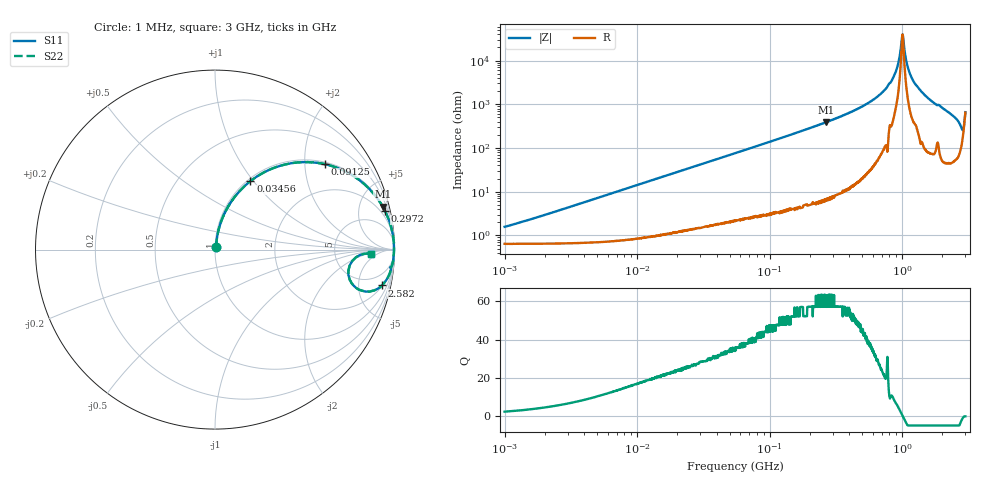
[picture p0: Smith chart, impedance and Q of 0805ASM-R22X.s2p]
!s-Parameter Generated by FASTRON Sdn. Bhd.
!FASTRON P/N : 0805ASM-R22X
!Keysight Technologies: E4991B_MY54100416_A.01.15
!Date: Fri Jun 19 14:51:07 2026
!Version  :Rev00  Fri Jun 19 14:51:07 2026
!Data & Calibration Information:
!Freq  S11  S21  S12  S22
!PortZ  Port1:50+j0  Port2:50+j0
!When reading reference impedance value at option line is always used.
! Remarks : This data is being provided solely for informational purposes.
# Hz S dB R 50
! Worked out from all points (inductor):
!   1601 points, 1 MHz to 3 GHz, reference 50 ohm
!   read as one part in series: L = 228 nH near 1.35 MHz
!   highest Q = 63.3 at 267.6 MHz (marker M1), where L = 234 nH
!   self-resonance near 1.003 GHz
!   S11 on the Smith chart (normalised r, x): 1 MHz: 1.01, +0.03; 34.56 MHz: 1.03, +0.96; 91.25 MHz: 1.06, +2.53; 297.2 MHz: 1.15, +8.84; 2.582 GHz: 2.10, -8.95; 3 GHz: 14, -3
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1000000  -36.10 65.1  -0.06 -0.8  -0.06 -0.8  -36.10 65.1
3804036  -25.30 79.9  -0.07 -3.1  -0.07 -3.1  -25.30 79.9
1.447069e7  -14.00 75.8  -0.26 -11.4  -0.26 -11.4  -14.00 75.8
3.456417e7  -7.35 62.7  -1.02 -25.4  -1.02 -25.4  -7.35 62.7
5.504702e7  -4.45 51.6  -2.11 -36.8  -2.11 -36.8  -4.45 51.6
9.124879e7  -2.21 37.8  -4.24 -50.9  -4.24 -50.9  -2.21 37.8
2.083556e8  -0.51 18.5  -9.96 -70.5  -9.96 -70.5  -0.51 18.5
2.675872e8  -0.31 14.3  -12.20 -74.8  -12.20 -74.8  -0.31 14.3
2.972367e8  -0.25 12.7  -13.20 -76.3  -13.20 -76.3  -0.25 12.7
5.611759e8  -0.06 5.2  -20.90 -83.3  -20.90 -83.3  -0.06 5.2
7.925923e8  -0.03 2.0  -29.30 -83.7  -29.30 -83.7  -0.03 2.0
8.982141e8  -0.02 1.0  -35.20 -80.3  -35.20 -80.3  -0.02 1.0
9.349007e8  -0.02 0.6  -38.80 -77.1  -38.80 -77.1  -0.02 0.6
9.828732e8  -0.02 0.2  -47.20 -55.5  -47.20 -55.5  -0.02 0.2
1.007775e9  -0.02 -0.0  -52.00 4.0  -52.00 4.0  -0.02 -0.0
1.033307e9  -0.02 -0.2  -46.60 57.0  -46.60 57.0  -0.02 -0.2
1.11944e9  -0.02 -0.9  -35.70 79.6  -35.70 79.6  -0.02 -0.9
1.255985e9  -0.04 -1.9  -29.30 81.3  -29.30 81.3  -0.04 -1.9
1.629261e9  -0.07 -4.5  -22.10 82.1  -22.10 82.1  -0.07 -4.5
2.581816e9  -0.43 -12.1  -13.50 70.8  -13.50 70.8  -0.43 -12.1
2.825159e9  -1.70 -15.4  -10.40 46.5  -10.40 46.5  -1.70 -15.4
3e9  -1.20 -1.6  -17.60 10.7  -17.60 10.7  -1.20 -1.6
